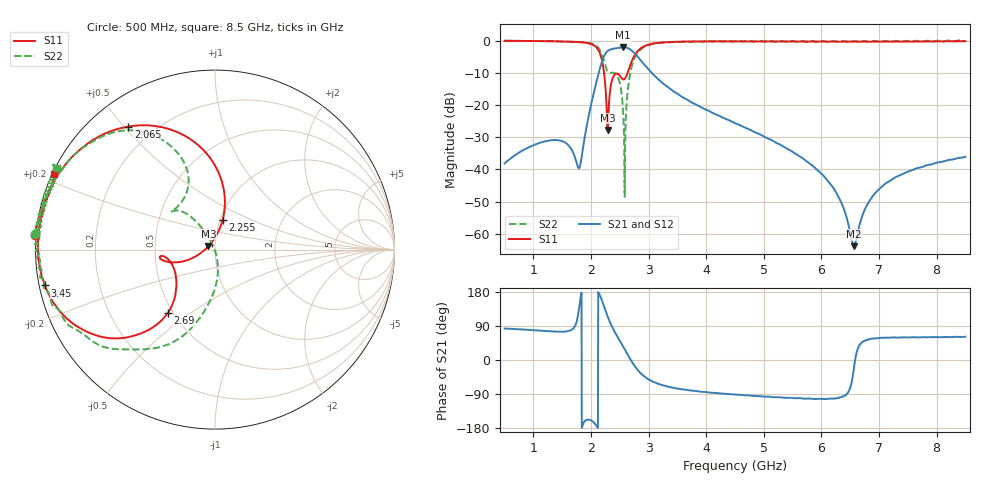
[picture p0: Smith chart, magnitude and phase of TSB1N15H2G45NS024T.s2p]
! TSB1N15H2G45NS024T  S-PARAMETER MODEL  ( General Type )
! Model Generated by TAIYO YUDEN Corporation (https://www.yuden.co.jp/en/)
! Version 2.0
! TAIYO YUDEN Control No. 090728
! Copyright(c) 2009 TAIYO YUDEN CO.,LTD. All Rights Reserved.
! Products Name : Multilayer Ceramic Devices
! Characteristics :
!  Passband freq : 2400-2500MHz ( At Passband , Insertion Loss : 3.0dB , VSWR 2.2 ),
!  Attenuation : 22dB min at 1710-1910MHz 20dB min at 4800-5000MHz, Impedance : 50 ohm ,
!  Case Size : 1.0 x 0.5 / 0.039 x 0.02 [mm/inch] , Thickness : 0.33 / 0.013 [mm/inch]
!  (Conditions: Temperature = 25 degC , DC Bias Current/Voltage = 0A / 0V)
! External Node Assignments :
!  1  o---|-------|---o  2
!  |  BPF  |
! GND o---|-------|---o GND
! Frequency Range : 500MHz  -  8.5GHz  [ 1601 STEP ]
# MHz S RI R 50
! Freq[MHz].  S11 Real  S11 Imag  S21 Real  S21 Imag  S12 Real  S12 Imag  S22 Real  S22 Imag
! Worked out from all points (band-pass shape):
!   1601 points, 500 MHz to 8.5 GHz, reference 50 ohm
!   highest |S21| = -1.94 dB at 2.56 GHz (marker M1); lowest = -63.9 dB at 6.57 GHz (marker M2)
!   |S21| within 3 dB of the highest: 2.222 GHz to 2.814 GHz (591.8 MHz wide, 23.5 % of centre)
!   lowest |S11| = -27.7 dB at 2.29 GHz (marker M3), VSWR 1.09, Z = 46.5 + j1.84 ohm
!   |S11| at or under -10 dB: 2.227 GHz to 2.634 GHz (406.8 MHz wide, 16.7 % of centre)
!   |S22| runs from -48.5 to 0.2 dB; largest |S21 - S12| = 0.0012
!   S11 on the Smith chart (normalised r, x): 500 MHz: -0.00, +0.04; 2.065 GHz: 0.11, +0.51; 2.255 GHz: 1.03, +0.35; 2.69 GHz: 0.47, -0.41; 3.45 GHz: 0.02, -0.10; 8.5 GHz: 0.00, +0.22
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500  -1.004 0.0833  0.00151 0.0123  0.00149 0.0123  -1.004 0.0895
1335  -0.9559 0.2572  0.00722 0.0278  0.00721 0.0278  -0.9548 0.2611
1835  -0.8201 0.491  -0.0151 0.00062  -0.0151 0.000623  -0.8379 0.4656
2065  -0.4828 0.6858  -0.1765 -0.0387  -0.1762 -0.0387  -0.5784 0.6491
2185  -0.0364 0.5228  -0.4322 0.1636  -0.4324 0.1632  -0.2516 0.5815
2255  0.0425 0.1644  -0.4073 0.4982  -0.4075 0.4981  -0.147 0.3714
2290  -0.0363 0.0198  -0.2895 0.6356  -0.29 0.6357  -0.1742 0.2843
2380  -0.2597 -0.0686  0.0893 0.7502  0.0889 0.7501  -0.2429 0.212
2480  -0.2986 -0.0355  0.4378 0.6497  0.437 0.6502  -0.1591 0.2001
2560  -0.2345 -0.0928  0.6551 0.4595  0.6552 0.4594  -0.0331 0.0635
2605  -0.2156 -0.1701  0.7307 0.3078  0.7307 0.3078  0.0131 -0.0638
2690  -0.2634 -0.3533  0.7287 0.000148  0.7292 0.000272  -0.058 -0.3409
2845  -0.557 -0.4947  0.4416 -0.2803  0.4415 -0.2802  -0.4442 -0.5566
3170  -0.8765 -0.3278  0.1147 -0.2268  0.1148 -0.2266  -0.8508 -0.3696
3450  -0.9484 -0.1999  0.0451 -0.1543  0.0452 -0.1542  -0.9453 -0.227
4500  -0.9855 0.0583  -0.00094 -0.0525  -0.000949 -0.0526  -0.9845 0.0693
5835  -0.9424 0.2717  -0.00245 -0.0114  -0.00245 -0.0114  -0.9597 0.2832
6280  -0.9212 0.3229  -0.000737 -0.00393  -0.000728 -0.00392  -0.9136 0.3346
6570  -0.9114 0.3503  0.000618 -0.000169  0.000632 -0.00017  -0.9276 0.3723
6795  -0.9042 0.3712  0.00169 0.00226  0.0017 0.00226  -0.9036 0.386
7170  -0.8955 0.3962  0.00338 0.00555  0.00338 0.00557  -0.8873 0.4132
8500  -0.8984 0.423  0.0075 0.0138  0.00749 0.0138  -0.8807 0.4571
